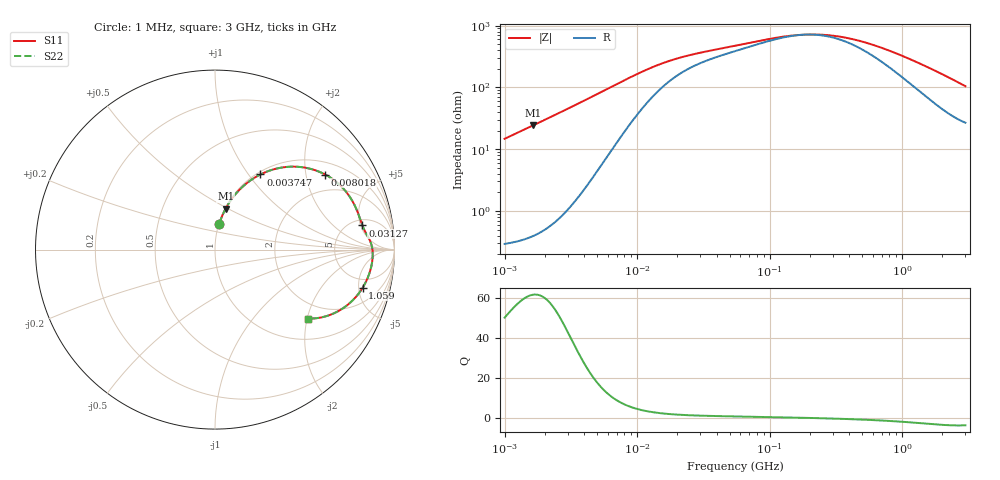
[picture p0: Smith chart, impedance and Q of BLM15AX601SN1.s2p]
! BLM15AX601SN1
# Hz S RI R 50
!Freq.(Hz) S11(Real) S11(Imag) S21(Real) S21(Imag) S12(Real) S12(Imag) S22(Real) S22(Imag)
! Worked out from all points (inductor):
!   401 points, 1 MHz to 3 GHz, reference 50 ohm
!   read as one part in series: L = 2.35 uH near 1.041 MHz
!   highest Q = 61.7 at 1.649 MHz (marker M1), where L = 2.36 uH
!   self-resonance near 184.5 MHz
!   S11 on the Smith chart (normalised r, x): 1 MHz: 1.01, +0.29; 3.747 MHz: 1.04, +1.14; 8.018 MHz: 1.38, +2.58; 31.27 MHz: 6.13, +5.37; 1.059 GHz: 3.65, -5.56; 3 GHz: 1.54, -2.02
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1000000  0.024 0.1433  0.976 -0.1433  0.976 -0.1433  0.024 0.1433
1649378  0.0596 0.2287  0.9404 -0.2287  0.9404 -0.2287  0.0596 0.2287
2561897  0.133 0.33  0.867 -0.33  0.867 -0.33  0.133 0.33
3747356  0.2534 0.4189  0.7466 -0.4189  0.7466 -0.4189  0.2534 0.4189
3823119  0.2615 0.4228  0.7385 -0.4228  0.7385 -0.4228  0.2615 0.4228
5592179  0.4413 0.4622  0.5587 -0.4622  0.5587 -0.4622  0.4413 0.4622
8017732  0.614 0.4183  0.386 -0.4183  0.386 -0.4183  0.614 0.4183
1.061086e7  0.7094 0.346  0.2906 -0.346  0.2906 -0.346  0.7094 0.346
1.461624e7  0.7706 0.2613  0.2294 -0.2613  0.2294 -0.2613  0.7706 0.2613
2.095589e7  0.8025 0.1881  0.1975 -0.1881  0.1975 -0.1881  0.8025 0.1881
3.127247e7  0.8211 0.1349  0.1789 -0.1349  0.1789 -0.1349  0.8211 0.1349
5.477226e7  0.8435 0.0877  0.1565 -0.0877  0.1565 -0.0877  0.8435 0.0877
1.244416e8  0.8711 0.0294  0.1289 -0.0294  0.1289 -0.0294  0.8711 0.0294
2.094008e8  0.8782 -0.00985  0.1218 0.00985  0.1218 0.00985  0.8782 -0.00985
2.884452e8  0.8786 -0.0365  0.1214 0.0365  0.1214 0.0365  0.8786 -0.0365
3.973271e8  0.8757 -0.0672  0.1243 0.0672  0.1243 0.0672  0.8757 -0.0672
5.473095e8  0.8684 -0.1043  0.1316 0.1043  0.1316 0.1043  0.8684 -0.1043
8.005644e8  0.8495 -0.1605  0.1505 0.1605  0.1505 0.1605  0.8495 -0.1605
1.059487e9  0.8231 -0.2118  0.1769 0.2118  0.1769 0.2118  0.8231 -0.2118
1.782824e9  0.7204 -0.3219  0.2796 0.3219  0.2796 0.3219  0.7204 -0.3219
2.359433e9  0.6228 -0.37  0.3772 0.37  0.3772 0.37  0.6228 -0.37
3e9  0.5181 -0.3843  0.4819 0.3843  0.4819 0.3843  0.5181 -0.3843
